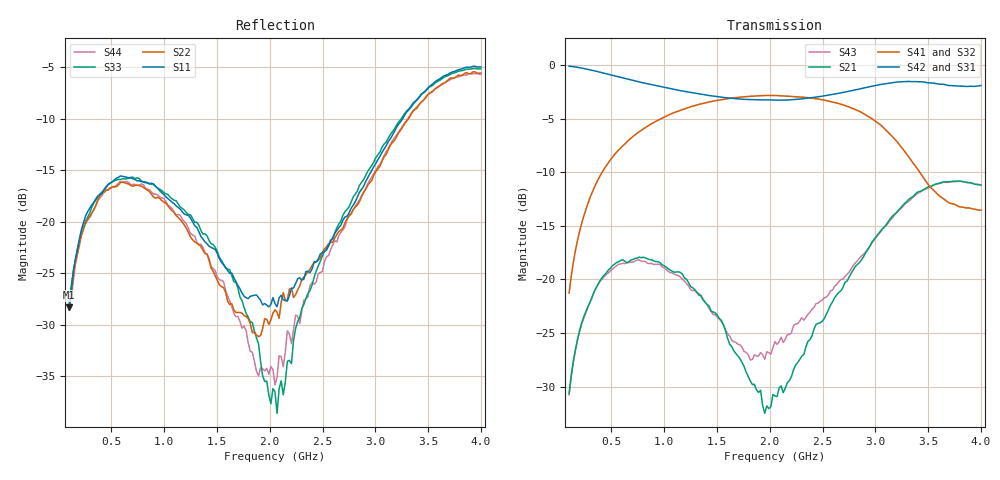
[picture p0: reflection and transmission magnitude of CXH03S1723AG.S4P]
!Agilent Technologies,E5071C,MY46418356,A.11.36
!Date: Mon Aug 05 11:41:45 2024
!Data & Calibration Information:
!Freq	S11:SOLT4(ON)	S12:SOLT4(ON)	S13:SOLT4(ON)	S14:SOLT4(ON)
!	S21:SOLT4(ON)	S22:SOLT4(ON)	S23:SOLT4(ON)	S24:SOLT4(ON)
!	S31:SOLT4(ON)	S32:SOLT4(ON)	S33:SOLT4(ON)	S34:SOLT4(ON)
!	S41:SOLT4(ON)	S42:SOLT4(ON)	S43:SOLT4(ON)	S44:SOLT4(ON)
!PortZ  Port1:50+j0  Port2:50+j0  Port3:50+j0  Port4:50+j0
!Above PortZ is port z conversion or system Z0 setting when saving the data.
!When reading, reference impedance value at option line is always used.
# Hz S dB R 50
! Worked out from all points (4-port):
!   201 points, 100 MHz to 4 GHz, reference 50 ohm
!   strongest paths, dB at 100 MHz, 1.075 GHz, 2.05 GHz, 3.025 GHz, 4 GHz:
!     S42: -0.1, -2.2, -3.3, -1.9, -1.9
!     S31: -0.1, -2.3, -3.2, -1.8, -1.9
!     S41: -21.3, -4.5, -2.8, -5.4, -13.5
!     S32: -21.3, -4.5, -2.9, -5.4, -13.3
!     S21: -30.6, -19.2, -30.9, -15.8, -11.2
!     S43: -30.8, -19.4, -25.8, -15.9, -11.2
!   lowest |S11| = -28.3 dB at 100 MHz (marker M1), VSWR 1.08, Z = 49.4 - j3.78 ohm
!   |S11| at or under -10 dB: start of sweep to 3.258 GHz
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1e8  -28.31 -96.7  -30.56 77.2  -0.08 -8.0  -21.27 80.8
     -30.64 77.3  -28.56 -100.2  -21.26 80.9  -0.09 -7.8
     -0.10 -7.9  -21.28 81.0  -27.96 -103.3  -30.73 76.7
     -21.27 80.8  -0.09 -7.8  -30.78 76.5  -28.14 -101.3
3.925e8  -17.35 -127.3  -20.13 35.1  -0.66 -28.9  -10.34 58.3
         -20.13 34.8  -17.45 -127.5  -10.35 58.5  -0.67 -28.4
         -0.68 -28.9  -10.36 58.5  -17.29 -130.0  -20.19 34.2
         -10.35 58.2  -0.66 -28.4  -20.18 34.0  -17.66 -127.3
8.995e8  -16.31 -166.3  -18.27 -21.7  -1.89 -58.2  -5.36 30.0
         -18.27 -22.2  -17.58 -166.1  -5.34 30.5  -1.85 -57.1
         -1.90 -58.1  -5.36 30.6  -16.39 -165.7  -18.69 -18.7
         -5.36 30.0  -1.85 -57.1  -18.59 -18.8  -17.31 -167.0
1.621e9  -25.00 142.4  -26.07 -68.0  -3.08 -92.3  -3.12 -1.8
         -26.05 -68.6  -28.04 142.8  -3.09 -0.9  -3.08 -90.4
         -3.10 -92.2  -3.11 -0.8  -24.65 164.8  -25.42 -53.8
         -3.10 -1.9  -3.08 -90.4  -25.28 -54.1  -27.70 150.6
2.0695e9  -28.25 70.0  -30.76 -17.7  -3.22 -111.5  -2.85 -20.4
          -30.93 -20.6  -28.78 67.4  -2.83 -19.1  -3.27 -109.1
          -3.24 -111.4  -2.86 -19.0  -38.61 65.1  -26.06 -23.5
          -2.84 -20.4  -3.26 -109.1  -26.07 -24.3  -35.08 44.9
3.0055e9  -14.31 -45.2  -16.09 -23.1  -1.85 -158.7  -5.28 -61.1
          -16.06 -23.3  -15.09 -33.2  -5.26 -59.1  -1.91 -154.5
          -1.86 -158.5  -5.27 -59.0  -13.74 -51.7  -16.16 -36.3
          -5.26 -61.1  -1.89 -154.5  -16.08 -36.5  -14.96 -50.5
4e9  -4.94 -129.5  -11.20 -134.4  -1.91 137.9  -13.59 -28.6
     -11.20 -134.3  -5.54 -125.5  -13.23 -28.2  -1.93 142.1
     -1.93 138.2  -13.27 -28.1  -5.13 -139.8  -11.28 -145.0
     -13.53 -28.4  -1.90 142.0  -11.21 -145.4  -5.68 -135.9
